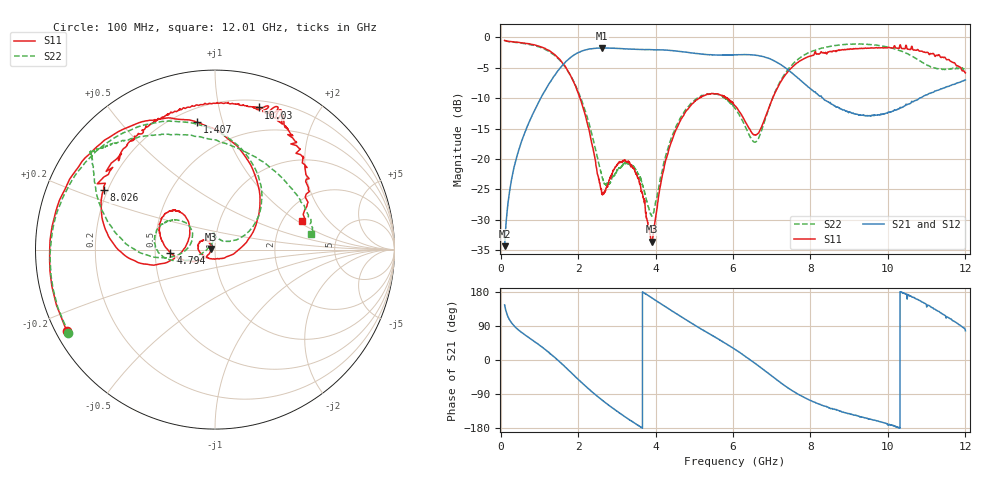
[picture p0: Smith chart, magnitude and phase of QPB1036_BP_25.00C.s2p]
! TDS: K:\Engsetup\Winsaw\QPB1036_ALL
! Channel 1
! Ports=1 2
! seg 1=100.000000 1100.000000 101
! seg 2=1101.000000 1501.000000 401
! seg 3=1502.000000 2502.000000 101
! seg 4=2503.000000 3803.000000 1301
! seg 5=3804.000000 5004.000000 121
! seg 6=5005.000000 6005.000000 1001
! seg 7=6006.000000 8406.000000 241
! seg 8=8407.000000 10607.000000 2201
! seg 9=10608.000000 12008.000000 141
! Points=5609
! FailCode=0
! Topology=ALL_SE(12)
!VNA Cal loaded =QPB1036_ALL_25C
!PS1(V)= 5.000
!PS(mA)= 0.700
!PS2(V)= 1.170
!PS(mA)= -0.100
!PS3(V)= 1.170
!PS(mA)= 0.100
!PS4(V)= 1.170
!PS(mA)= -0.100
!Temp (C)= 25.00
# MHz S DB R 50
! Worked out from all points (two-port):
!   5609 points, 100 MHz to 12.01 GHz, reference 50 ohm
!   highest |S21| = -1.74 dB at 2.611 GHz (marker M1); lowest = -34.3 dB at 100 MHz (marker M2)
!   |S21| within 3 dB of the highest: 1.575 GHz to 7.295 GHz (5.721 GHz wide, 129 % of centre)
!   lowest |S11| = -33.6 dB at 3.904 GHz (marker M3), VSWR 1.04, Z = 48 + j0.312 ohm
!   |S11| at or under -10 dB: 2.049 GHz to 5.136 GHz (3.087 GHz wide, 85.9 % of centre); 5.845092 GHz to 5.846803 GHz (1.711 MHz wide, 0.0293 % of centre); 5.85 GHz to 7.027 GHz (1.177 GHz wide, 18.3 % of centre)
!   |S22| runs from -29.4 to -0.5 dB; largest |S21 - S12| = 0.12
!   S11 on the Smith chart (normalised r, x): 100 MHz: 0.03, -0.26; 1.407 GHz: 0.29, +0.83; 4.794 GHz: 0.60, -0.02; 8.026 GHz: 0.18, +0.24; 10.03 GHz: 0.26, +1.32; 12.01 GHz: 2.54, +1.10
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100  -0.52 -151.3  -34.33 145.3  -34.29 145.9  -0.54 -150.5
730  -1.05 144.7  -13.99 58.7  -13.99 58.6  -1.18 148.2
1407  -2.91 97.8  -6.15 5.9  -6.11 5.9  -3.06 97.6
2092  -10.84 34.9  -2.26 -59.8  -2.28 -59.6  -10.37 37.2
2611  -25.74 -73.2  -1.74 -105.1  -1.76 -105.4  -22.61 40.8
3309  -20.65 151.7  -1.91 -156.6  -1.93 -156.5  -20.78 94.4
3793  -30.32 130.6  -2.01 171.3  -2.02 171.4  -27.46 109.4
3904  -33.60 171.1  -2.02 164.2  -2.02 163.8  -29.41 142.9
4074  -26.32 -142.4  -2.05 152.6  -2.03 152.6  -25.09 -172.0
4794  -12.08 -175.7  -2.45 105.6  -2.44 105.7  -11.77 -167.2
5455  -9.22 149.9  -2.89 65.3  -2.86 65.3  -9.26 166.7
6056  -11.28 132.2  -2.88 27.9  -2.84 27.6  -11.69 141.1
6586  -16.09 162.2  -2.94 -9.9  -2.94 -9.9  -17.18 163.6
7116  -8.76 -166.4  -4.02 -51.2  -4.03 -51.1  -8.64 -174.7
8026  -3.06 151.9  -8.55 -107.7  -8.52 -108.1  -2.35 151.1
8046  -2.95 150.9  -8.68 -108.8  -8.66 -109.0  -2.27 150.8
8961  -1.96 109.6  -12.18 -141.0  -12.17 -140.3  -1.14 142.3
10024  -1.64 73.1  -12.29 -171.0  -12.37 -168.6  -1.66 134.6
10026  -1.64 73.0  -12.28 -171.0  -12.36 -168.7  -1.67 134.6
10928  -2.43 57.8  -9.66 151.3  -9.71 150.9  -4.25 91.8
11498  -3.46 40.7  -8.23 116.4  -8.21 116.2  -5.24 37.7
12008  -5.85 18.3  -7.01 77.2  -7.08 85.7  -5.29 8.2
